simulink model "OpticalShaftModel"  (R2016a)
settings: Solver=VariableStepAuto  StartTime=0.0  StopTime=10.0  RelTol=1e-3
libraries: vexarmcortexlib x2

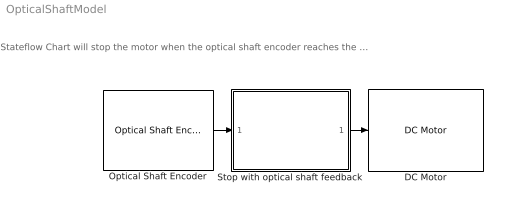
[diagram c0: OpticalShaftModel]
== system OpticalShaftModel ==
  note: Stateflow Chart will stop the motor when the optical shaft encoder reaches the set-point
  DC Motor : vexarmcortexlib/DC Motor  motor=7  scaleFactor=1/13.5  SimulationOut=off
  Optical Shaft Encoder : vexarmcortexlib/Optical Shaft Encoder  topPort=11  bottomPort=12  resetOption=No reset  inputPortSim=off  SampleTime=0.2
  Stop with optical shaft feedback : Stateflow chart  TreatAsAtomicUnit=on
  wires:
  Stop with optical shaft feedback/1(speed) -> DC Motor/1
  Optical Shaft Encoder/1 -> Stop with optical shaft feedback/1(shaft)

== stateflow chart OpticalShaftModel/Stop with optical shaft 
feedback ==
  state <!DOCTYPE HTML PUBLIC "-//W3C//DTD HTML 4.0//EN" "http://www.w3.org/TR/REC-html40/strict.dtd"> [group]
    <html><head><meta name="qrichtext" content="1" /><style type="text/css">
    p, li { white-space: pre-wrap; }
    </style></head><body style=" font-family:'Helvetica'; font-size:12px; font-weight:400; font-style:normal;">
    <p style=" margin-top:0px; margin-bottom:0px; margin-left:0px; margin-right:0px; -qt-block-indent:0; text-indent:0px;">Stateflow Chart <span style=" font-style:italic;">transitions</span> to <span style=" font-weight:600;">Stop</span> when</p>
    <p style=" margin-top:0px; margin-bottom:0px; margin-left:0px; margin-right:0px; -qt-block-indent:0; text-indent:0px;">the value of the input variable <span style=" font-style:italic;">shaft</span> </p>
    <p style=" margin-top:0px; margin-bottom:0px; margin-left:0px; margin-right:0px; -qt-block-indent:0; text-indent:0px;">reaches 360 ticks or degrees</p></body></html>
  state Drive_Forward
    during:
    speed = 30;
  state Stop
    during:
    speed =0;
  (default) -> Drive_Forward : {speed = 0;}
  Drive_Forward -> Stop : [shaft > 360]
  data: shaft input; speed output
